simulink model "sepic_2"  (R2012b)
settings: Solver=ode45  StartTime=0.0  StopTime=10.0  RelTol=1e-3
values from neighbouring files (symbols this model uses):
  C1 = 200e-6    (= 0.0002)    [Cuk1.m]    (also in sepic1.m = 0.0001; sepic2.m = 0.0001; feder_masse_1.m = [1 0 0 0]; feder_masse_13.m = [1 0 0 0])
  C2 = C1    (= 0.0002)    [Cuk1.m]    (also in sepic1.m = 0.0001; sepic2.m = 0.0001; feder_masse_1.m = [0 0 1 0]; feder_masse_13.m = [0 0 1 0])
  f0 = 0.2e5    (= 20000)    [boost_up1.m]    (also in buck_boost1.m; buck_boost2.m; buck_down1.m; buck_down2.m)
  L1 = 0.0001    [Cuk1.m]    (also in sepic1.m = 5e-05; sepic2.m = 5e-05)
  L2 = L1    (= 0.0001)    [Cuk1.m]    (also in sepic1.m = 5e-05; sepic2.m = 5e-05)
  M = 0.8*L1    (= 4e-05)    [sepic2.m]    (also in rad_aufhaeng_1.m = [ms 0;0 ma]; rad_aufhaeng_2.m = [ms 0;0 ma]; rad_aufhaeng_3.m = [ms 0;0 ma]; rad_aufhaeng_4.m = [ms 0;0 ma])
  R = 5    [boost_up1.m]    (also in buck_boost1.m; buck_boost2.m; buck_down1.m = 2*Rmax,; buck_down2.m = 0.1*Rmax,)
  T = 1/f0    (= 5e-05)    [boost_up1.m]    (also in buck_boost1.m; buck_boost2.m; buck_down1.m; buck_down2.m)
  T1 = T-T2    (= 2.5e-05)    [buck_boost1.m]    (also in buck_boost2.m = 1e-05; sepic1.m = T-T2; sepic2.m = T-T2; unwucht_4.m = 500)
  Ui = 5    [boost_up1.m]    (also in buck_boost1.m; buck_boost2.m; buck_down1.m; buck_down2.m)

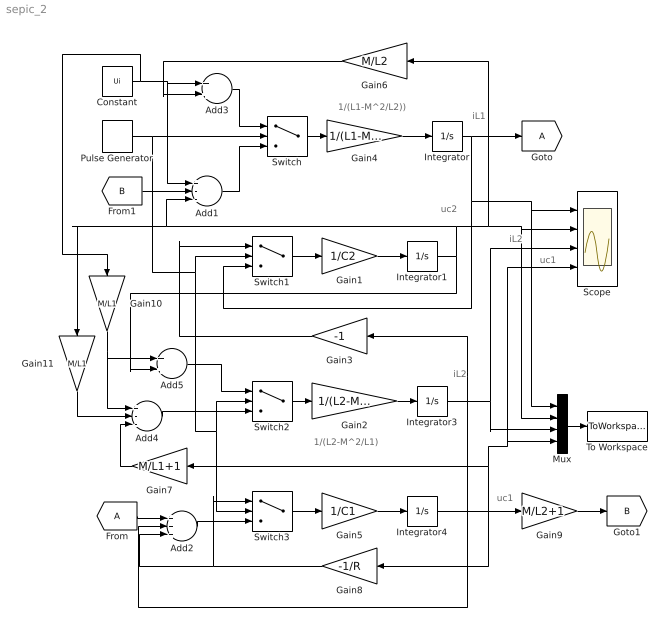
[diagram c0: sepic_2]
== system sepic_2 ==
  note: 1/(L2-M^2/L1)
  note: 1/(L1-M^2/L2))
  note: uc1
  note: iL2
  note: uc1
  note: iL2
  note: uc2
  note: iL1
  Add1 : Sum  Inputs=+--
  Add2 : Sum  Inputs=+++
  Add3 : Sum
  Add4 : Sum  Inputs=+--
  Add5 : Sum
  Constant : Constant  Value=Ui
  From : From
  Gain1 : Gain  Gain=1/C2
  Gain10 : Gain  Gain=M/L1
  Gain11 : Gain  Gain=M/L1
  Gain2 : Gain  Gain=1/(L2-M^2/L1)
  Gain3 : Gain  Gain=-1
  Gain4 : Gain  Gain=1/(L1-M^2/L2)
  Gain5 : Gain  Gain=1/C1
  Gain6 : Gain  Gain=M/L2
  Gain7 : Gain  Gain=M/L1+1
  Gain8 : Gain  Gain=-1/R
  Gain9 : Gain  Gain=M/L2+1
  Integrator{,1,3..4} (4 alike) : Integrator
  Mux : Mux
  Pulse Generator : DiscretePulseGenerator  PulseType=Time based  Period=1/f0  PulseWidth=T1*100/T
  Scope : Scope  NumInputPorts=4
  Switch{,1..3} (4 alike) : Switch  Criteria=u2 > Threshold  Threshold=0.5  ZeroCross=off  SampleTime=0
  To Workspace : ToWorkspace  VariableName=y  SampleTime=-1  SaveFormat=Structure With Time
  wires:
  Pulse Generator/1 -> Switch/2, Switch3/2, Switch2/2, Switch1/2
  Add1/1 -> Switch/3
  Switch/1 -> Gain4/1
  Gain4/1 -> Integrator/1
  Switch1/1 -> Gain1/1
  Gain1/1 -> Integrator1/1
  Switch2/1 -> Gain2/1
  Gain2/1 -> Integrator3/1
  Integrator/1 -> Mux/1, Scope/1, Switch1/3, [A]
  Add4/1 -> Switch2/3
  Mux/1 -> To Workspace/1
  Switch3/1 -> Gain5/1
  Gain5/1 -> Integrator4/1
  Add2/1 -> Switch3/3
  From/1 -> Add2/1
  Integrator3/1 -> Add2/2, Gain3/1, Mux/3, Scope/3
  Integrator4/1 -> Gain9/1, Scope/4, Mux/4, Gain7/1, Gain8/1
  Gain8/1 -> Add2/3, Switch3/1
  [B] -> Add1/2
  Gain3/1 -> Switch1/1
  Add3/1 -> Switch/1
  Gain6/1 -> Add3/2
  Gain9/1 -> [B]
  Constant/1 -> Gain10/1, Add3/1, Add1/1
  Gain7/1 -> Add4/3
  Gain10/1 -> Add4/1, Add5/1
  Add5/1 -> Switch2/1
  Integrator1/1 -> Add5/2, Gain11/1, Add1/3, Gain6/1, Mux/2, Scope/2
  Gain11/1 -> Add4/2
